TYPE IDENTControl_UserData :
STRUCT	
	ReadData:			ARRAY[0..245] OF BYTE;	(* Read in data from data carrier*)	
	WriteData:			ARRAY[0..245] OF BYTE;	(* Write data to data carrier *)
	SpecialCommand:		ARRAY[0..30] OF BYTE;	(* Bypass for commands, which are not included in FB *)
	ReadParam_IF:		BYTE;					(* Parameter IF; information frame with RSSI; only MultiFrame; Default = 16#00; 16#00 = switched off; 16#01 = switched on*)
	ReadParam_AF:		BYTE;					(* Parameter AF; AFI to request; Default = 16#00 all tags*)
	ReadParam_E5 : 		BYTE;					(* Parameter E5; Tag Lost smoothing; Default = 16#05*)
	ReadParam_NT : 		BYTE;					(* Parameter NT; Number of Tags to find; Default = 16#FF*)
	ReadParam_QV : 		BYTE;					(* Parameter QV; Protocol Mode; Default = 16#53 SingleFrame Protocol*)
	ReadParam_QW : 		BYTE;					(* Parameter QW; Definition of used Time slots; Default = 16#00*)
	ReadParam_TA : 		BYTE;					(* Parameter TA; Tries allowed; Default = 16#02*)
	ReadParam_PT : 		WORD;					(* Parameter PT; Power setting; Default = 16#0004 Max*)
	ReadParam_DR : 		BYTE;					(* Parameter DR; Data rate for read; Default 16#00*)
	ReadParam_TI:		ARRAY[0..9] OF BYTE;	(* Parameter TI; Filter for Tag UID; Default = no filter*)
	ReadParam_TO : 		BYTE;					(* Parameter TO; Overtemperature handling; Default = 16#00*)
	ReadParam_CT:		INT;					(* Parameter CT; TagType; Default = 20(dec)*)
	ReadParam_OH:		ARRAY[0..5] OF DWORD;	(* Parameter OH; Operating Hours*)
	ReadParam_TE:		ARRAY[0..1] OF INT;		(* Parameter TE; Temperatures in C°*)
	ReadParam_VO:		ARRAY[0..9] OF UINT;	(* Parameter VO; Voltages / current in mV/mA*)
	ReadParam_FR:		BYTE;					(* Parameter FR; Sequence Mode; Default 16#01 (Write after Read)*)
	ReadParam_RV:		STRING[56];				(* Parameter RV; Read Version GIT*)
	ReadParam_SN:		ARRAY[0..11] OF BYTE;	(* Parameter SN; Read serial number of uC*)
	ReadParam_MM:		BYTE;					(* Parameter MM; MultiPlex Mode*)
	ReadParam_ST:		ARRAY[0..1] OF BYTE;	(* Parameter ST; Status of Frontend*)
	WriteParam_IF: 		BYTE := 16#00;			(* Parameter IF; information frame with RSSI; only MultiFrame; Default = 16#00; 16#00 = switched off; 16#01 = switched on*)
	WriteParam_AF: 		BYTE := 16#00;			(* Parameter AF; AFI to request; Default = 16#00 all tags*)
	WriteParam_E5:		BYTE := 16#05;			(* Parameter E5; Tag Lost smoothing; Default = 16#05*)
	WriteParam_NT:		BYTE := 16#FF;			(* Parameter NT; Number of Tags to find; Default = 16#FF*)
	WriteParam_QV:		BYTE := 16#53;			(* Parameter QV; Protocol Mode; Default = 16#53 SingleFrame Protocol*)
	WriteParam_QW:		BYTE := 16#00;			(* Parameter QW; Definition of used Time slots; Default = 16#00*)
	WriteParam_TA:		BYTE := 16#02;			(* Parameter TA; Tries allowed; Default = 16#02*)
	WriteParam_PT:		WORD := 16#0004;		(* Parameter PT; Power setting; Default = 16#0004 Max*)
	WriteParam_DR:		BYTE := 16#00;			(* Parameter DR; Data rate for read; Default 16#00*)
	WriteParam_TI:		ARRAY[0..9] OF BYTE;	(* Parameter TI; Filter for Tag UID; Default = no filter*)
	WriteParam_TO:		BYTE := 16#00;			(* Parameter TO; Overtemperature handling; Default = 16#00*)
	WriteParam_FR:		BYTE := 16#01;			(* Parameter FR; Sequence Mode; Default 16#01 (Write after Read)*)
END_STRUCT
END_TYPE
